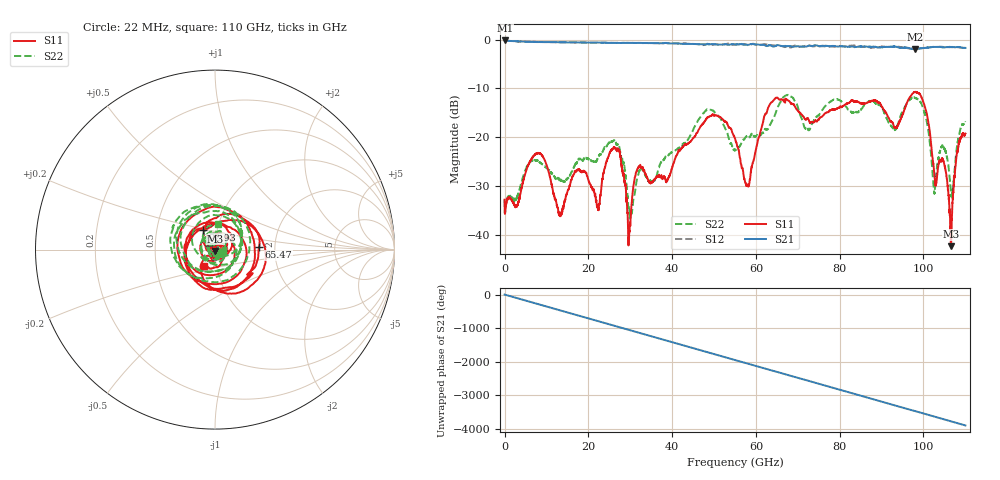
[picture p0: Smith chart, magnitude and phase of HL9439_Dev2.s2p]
! 4/1/2022 11:05:40 AM
! C:\USERS\VECTORSTARUSER\DESKTOP\JASON\100GDCB\AS21.S2P
! CHANNEL.1
! TR.MEASUREMENT
! CORRECTED.DATA
# GHZ S RI R 50.0
! FREQ.GHZ  S11RE  S11IM  S21RE  S21IM  S12RE  S12IM  S22RE  S22IM
!; PortSelection: Port_12
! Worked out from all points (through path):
!   5000 points, 22 MHz to 110 GHz, reference 50 ohm
!   highest |S21| = -0.14 dB at 66 MHz (marker M1); lowest = -1.9 dB at 98.05 GHz (marker M2)
!   group delay of S21, straight-line fit = 98.3 ps
!   lowest |S11| = -42.4 dB at 106.6 GHz (marker M3), VSWR 1.02, Z = 50.3 - j0.716 ohm
!   |S11| at or under -10 dB: start of sweep to end of sweep
!   |S22| runs from -36.7 to -11.3 dB; largest |S21 - S12| = 0.041
!   S11 on the Smith chart (normalised r, x): 22 MHz: 1.03, -0.03; 65.47 GHz: 1.65, +0.06; 92.93 GHz: 0.86, +0.19; 110 GHz: 0.86, -0.15
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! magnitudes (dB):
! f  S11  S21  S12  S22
! 22 MHz  -32.8  -0.2  -0.2  -32.8
! 66 MHz  -35.5  -0.1  -0.1  -35.6
! 7.656 GHz  -23.3  -0.4  -0.4  -24.8
! 13.29 GHz  -36.2  -0.5  -0.5  -28.8
! 18.37 GHz  -27.0  -0.5  -0.6  -24.8
! 22.35 GHz  -34.9  -0.6  -0.6  -24.0
! 26.97 GHz  -22.4  -0.7  -0.6  -21.5
! 29.77 GHz  -39.2  -0.6  -0.6  -34.6
! 31.9 GHz  -26.3  -0.6  -0.7  -27.8
! 36.7 GHz  -28.2  -0.7  -0.7  -26.7
! 48.53 GHz  -15.9  -0.9  -0.8  -14.3
! 55.02 GHz  -20.3  -1.0  -1.0  -22.7
! 58.06 GHz  -29.9  -1.0  -1.1  -19.8
! 65.47 GHz  -12.2  -1.1  -1.3  -13.4
! 73.35 GHz  -16.8  -1.3  -1.3  -17.4
! 91.67 GHz  -16.0  -1.5  -1.5  -17.0
! 92.93 GHz  -17.8  -1.4  -1.3  -18.6
! 98.05 GHz  -10.7  -1.9  -1.9  -11.9
! 102.5 GHz  -26.8  -1.5  -1.5  -31.2
! 104.7 GHz  -24.6  -1.6  -1.5  -21.9
! 106.6 GHz  -42.4  -1.5  -1.5  -31.4
! 110 GHz  -19.2  -1.7  -1.7  -17.0
